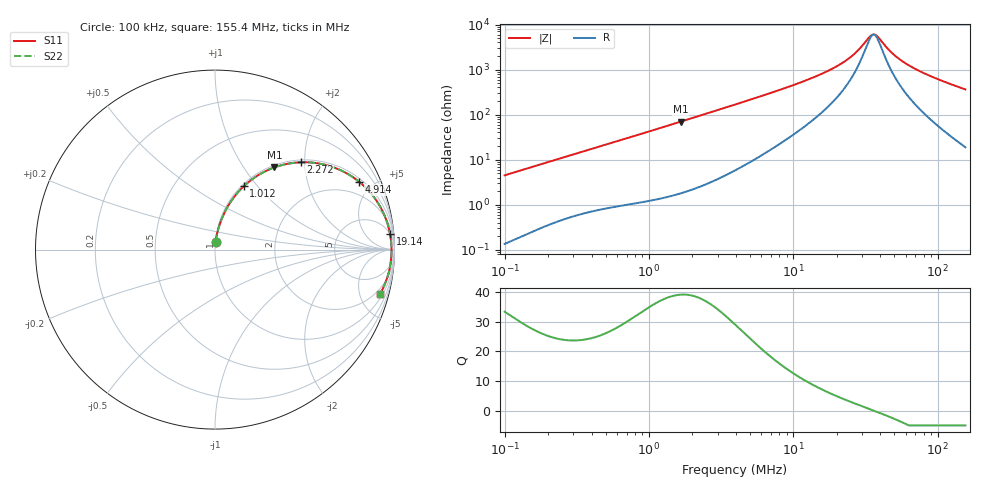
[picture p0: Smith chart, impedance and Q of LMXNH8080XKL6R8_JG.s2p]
! LMXNH8080XKL6R8_JG  S-PARAMETER MODEL  ( General Type )
! Model Generated by TAIYO YUDEN Corporation (http://www.ty-top.com)
! Version 1.0
! TAIYO YUDEN Control No. 191025NI43SB-FBB
! Copyright(c) 2019 TAIYO YUDEN CO.,LTD. All Rights Reserved.
! Product Description (link to TY-COMPAS)
! https://ds.yuden.co.jp/TYCOMPAS/or/detail?pn=LMXNH8080XKL6R8MJG&u=M
! Products Name : Inductors
! Characteristics :
!  Inductance : 6.8 uH , SRF(min) : 32 MHz , DC Resistance(max) : 0.0377 Ohm
!  Rated Current : Saturation :3000 mA , Temp Rise : 3400 mA
!  Case Size : 8.0 x 8.0 / 0.315 x 0.315 [mm/inch] , Thickness : 3 / 0.118 [mm/inch]
!  (Conditions: Temperature = 25 degC , DC Bias Current/Voltage = 0A / 0V)
! External Node Assignments :
!  1  o---GGG---o  2
! GND o---------o GND
! Frequency Range : 0.1MHz  -  155.401204MHz  [ 402 STEP ]
# MHz S RI R 50
! Freq[MHz].  S11 Real  S11 Imag  S21 Real  S21 Imag  S12 Real  S12 Imag  S22 Real  S22 Imag
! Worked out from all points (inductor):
!   401 points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, 100 kHz to 155.4 MHz, reference 50 ohm
!   read as one part in series: L = 7.08 uH near 103.7 kHz
!   highest Q = 39.1 at 1.662 MHz (marker M1), where L = 6.67 uH
!   self-resonance near 35.98 MHz
!   S11 on the Smith chart (normalised r, x): 100 kHz: 1.00, +0.09; 1.012 MHz: 1.02, +0.85; 2.272 MHz: 1.05, +1.91; 4.914 MHz: 1.17, +4.18; 19.14 MHz: 5, +22; 155.4 MHz: 1.38, -7.23
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0.1  0.00332 0.0445  0.9967 -0.0445  0.9967 -0.0445  0.00332 0.0445
0.342427  0.0271 0.1428  0.9729 -0.1428  0.9729 -0.1428  0.0271 0.1428
0.627861  0.0735 0.244  0.9265 -0.244  0.9265 -0.244  0.0735 0.244
1.012297  0.1604 0.353  0.8396 -0.353  0.8396 -0.353  0.1604 0.353
1.172566  0.2016 0.3879  0.7984 -0.3879  0.7984 -0.3879  0.2016 0.3879
1.662384  0.3312 0.4581  0.6688 -0.4581  0.6688 -0.4581  0.3312 0.4581
2.27179  0.4769 0.4864  0.5231 -0.4864  0.5231 -0.4864  0.4769 0.4864
3.942096  0.7283 0.428  0.2717 -0.428  0.2717 -0.428  0.7283 0.428
4.914404  0.8042 0.3771  0.1958 -0.3771  0.1958 -0.3771  0.8042 0.3771
7.779232  0.907 0.2614  0.093 -0.2614  0.093 -0.2614  0.907 0.2614
13.49882  0.9614 0.1441  0.0386 -0.1441  0.0386 -0.1441  0.9614 0.1441
19.13771  0.9756 0.0861  0.0244 -0.0861  0.0244 -0.0861  0.9756 0.0861
25.67722  0.9814 0.0442  0.0186 -0.0442  0.0186 -0.0442  0.9814 0.0442
33.20848  0.9835 0.0103  0.0165 -0.0103  0.0165 -0.0103  0.9835 0.0103
35.09012  0.9836 0.00323  0.0164 -0.00323  0.0164 -0.00323  0.9836 0.00323
36.40342  0.9837 -0.00152  0.0163 0.00152  0.0163 0.00152  0.9837 -0.00152
38.46609  0.9836 -0.00864  0.0164 0.00864  0.0164 0.00864  0.9836 -0.00864
46.22367  0.9828 -0.0327  0.0172 0.0327  0.0172 0.0327  0.9828 -0.0327
55.54574  0.9808 -0.0579  0.0192 0.0579  0.0192 0.0579  0.9808 -0.0579
71.83758  0.9751 -0.0963  0.0249 0.0963  0.0249 0.0963  0.9751 -0.0963
101.8464  0.9594 -0.1575  0.0406 0.1575  0.0406 0.1575  0.9594 -0.1575
155.4012  0.918 -0.2497  0.082 0.2497  0.082 0.2497  0.918 -0.2497
